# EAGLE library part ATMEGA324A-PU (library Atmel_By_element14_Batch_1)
8-bit Atmel Microcontroller
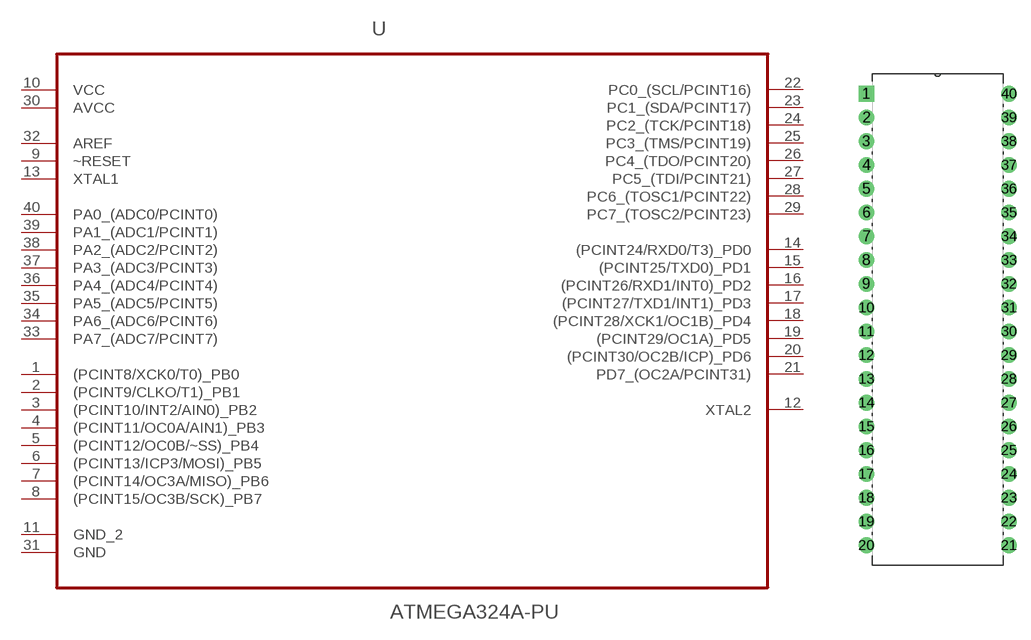
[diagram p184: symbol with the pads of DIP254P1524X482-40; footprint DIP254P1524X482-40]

Designator prefix U

## ATMEGA324A-PU (DESCRIPTION: 8-bit Atmel Microcontroller; MPN: ATMEGA324A-PU; OC_FARNELL: 1841611; OC_NEWARK: 68T2854; PACKAGE: DIP-40; SUPPLIER: Atmel)  [DIP254P1524X482-40]
1  (PCINT8/XCK0/T0)_PB0
2  (PCINT9/CLKO/T1)_PB1
3  (PCINT10/INT2/AIN0)_PB2
4  (PCINT11/OC0A/AIN1)_PB3
5  (PCINT12/OC0B/~SS)_PB4
6  (PCINT13/ICP3/MOSI)_PB5
7  (PCINT14/OC3A/MISO)_PB6
8  (PCINT15/OC3B/SCK)_PB7
9  ~RESET  in
10  VCC  pwr
11  GND_2  pas
12  XTAL2  out
13  XTAL1  in
14  (PCINT24/RXD0/T3)_PD0
15  (PCINT25/TXD0)_PD1
16  (PCINT26/RXD1/INT0)_PD2
17  (PCINT27/TXD1/INT1)_PD3
18  (PCINT28/XCK1/OC1B)_PD4
19  (PCINT29/OC1A)_PD5
20  (PCINT30/OC2B/ICP)_PD6
21  PD7_(OC2A/PCINT31)
22  PC0_(SCL/PCINT16)
23  PC1_(SDA/PCINT17)
24  PC2_(TCK/PCINT18)
25  PC3_(TMS/PCINT19)
26  PC4_(TDO/PCINT20)
27  PC5_(TDI/PCINT21)
28  PC6_(TOSC1/PCINT22)
29  PC7_(TOSC2/PCINT23)
30  AVCC  pwr
31  GND  pas
32  AREF  in
33  PA7_(ADC7/PCINT7)
34  PA6_(ADC6/PCINT6)
35  PA5_(ADC5/PCINT5)
36  PA4_(ADC4/PCINT4)
37  PA3_(ADC3/PCINT3)
38  PA2_(ADC2/PCINT2)
39  PA1_(ADC1/PCINT1)
40  PA0_(ADC0/PCINT0)

## Footprint DIP254P1524X482-40 (pad centres in mm)
drill 1.118 square: 1 -15.24,48.26
drill 1.118: 2 -15.24,45.72; 3 -15.24,43.18; 4 -15.24,40.64; 5 -15.24,38.1; 6 -15.24,35.56; 7 -15.24,33.02; 8 -15.24,30.48; 9 -15.24,27.94; 10 -15.24,25.4; 11 -15.24,22.86; 12 -15.24,20.32; 13 -15.24,17.78; 14 -15.24,15.24; 15 -15.24,12.7; 16 -15.24,10.16; 17 -15.24,7.62; 18 -15.24,5.08; 19 -15.24,2.54; 20 -15.24,0; 21 0,0; 22 0,2.54; 23 0,5.08; 24 0,7.62; 25 0,10.16; 26 0,12.7; 27 0,15.24; 28 0,17.78; 29 0,20.32; 30 0,22.86; 31 0,25.4; 32 0,27.94; 33 0,30.48; 34 0,33.02; 35 0,35.56; 36 0,38.1; 37 0,40.64; 38 0,43.18; 39 0,45.72; 40 0,48.26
